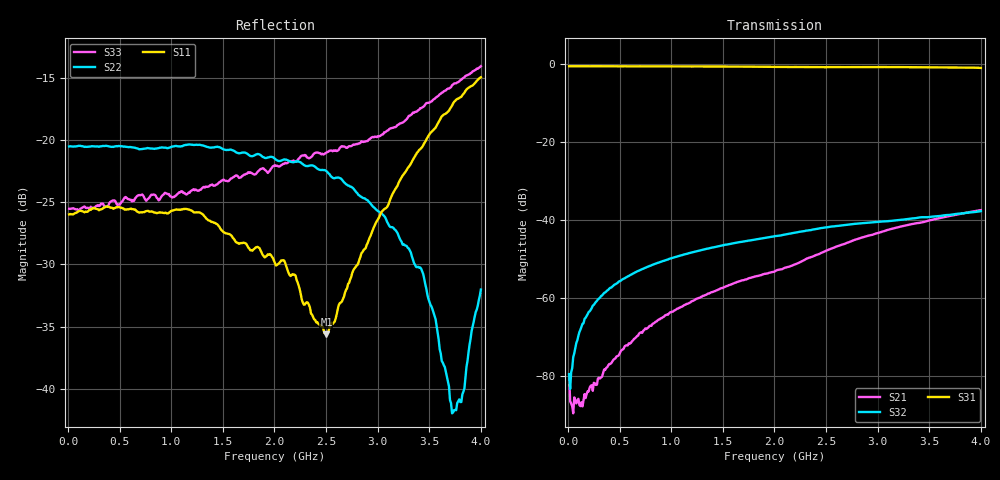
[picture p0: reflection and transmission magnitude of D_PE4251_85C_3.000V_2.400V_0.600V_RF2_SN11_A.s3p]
! Device ID: PE4251_SoldCshunt_081809
! Dir: c:\Test Bench Repositories\Bench_Software_CVI_Version_8\trunk\PSC 4Port_VNA Bench\datalog\4250\TEST\PE4251_SoldCshunt_081809\85C\3p000000\RF2
! Serial: 11
! Insertion: A
! Temp: 85C
! VDD: 3.000
! Control_Hi: 80.000
! Control_Lo: 20.000
! Logic State: RF2
! Port 1: RFC
! Port 2: RF1
! Port 3: RF2
! V1 = 0.60
! V2 = 0.60
! V3 = 0.60
! IDD: 4.342810e-05
! FILE NAME
! DATE 08/18/09  20:16
! CORRECTED  DATA
#  Hz  S  RI  R  50.00
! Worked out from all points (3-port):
!   401 points, 10 MHz to 4 GHz, reference 50 ohm
!   strongest paths, dB at 10 MHz, 1.008 GHz, 2.005 GHz, 3.002 GHz, 4 GHz:
!     S31: -0.6, -0.7, -0.8, -0.8, -1.1
!     S32: -79.4, -49.7, -44.1, -40.5, -37.7
!     S21: -79.6, -63.5, -53.1, -43.3, -37.5
!   lowest |S11| = -35.6 dB at 2.504 GHz (marker M1), VSWR 1.03, Z = 50.4 - j1.61 ohm
!   |S11| at or under -10 dB: start of sweep to end of sweep
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1e7  0.0502 -0.000826  9.81e-06 -2.35e-05  0.9306 -0.00374
     0.000105 6.75e-06  0.0942 -0.000936  2.63e-05 -3.63e-05
     0.931 -0.0045  1.43e-05 -0.000106  0.0529 0.000571
1.79575e8  0.0514 6.12e-05  7.43e-06 -5.77e-05  0.9288 -0.0635
           9.97e-06 -5.83e-05  0.0937 -0.00445  7.21e-05 0.00059
           0.9285 -0.0633  5.73e-05 0.00059  0.0533 -0.000987
3.19225e8  0.0526 -0.00155  -4.97e-05 -9.73e-05  0.9227 -0.1114
           -3.73e-05 -8.93e-05  0.0939 -0.00829  9.15e-05 0.00105
           0.9246 -0.1107  8.28e-05 0.00106  0.0554 -0.00304
4.888e8  0.0537 -0.00355  -0.000133 -0.00013  0.9126 -0.1684
         -0.000129 -0.000131  0.0938 -0.0121  0.000145 0.0016
         0.9129 -0.1676  0.000158 0.00161  0.0548 -0.00534
1.0075e9  0.0501 -0.0138  -0.000653 -0.000148  0.8626 -0.3352
          -0.000654 -0.000143  0.0902 -0.0264  0.000435 0.00324
          0.8638 -0.3354  0.000441 0.00325  0.0572 -0.0131
2.005e9  0.031 -0.00771  -0.00221 -6.32e-05  0.6873 -0.6014
         -0.00222 -4.25e-05  0.0772 -0.033  0.00103 0.00612
         0.6881 -0.6018  0.00102 0.00614  0.0691 -0.0387
2.50375e9  0.0046 -0.0159  -0.00404 -0.000364  0.5769 -0.6985
           -0.00406 -0.000383  0.0686 -0.0302  0.00136 0.00795
           0.579 -0.699  0.00137 0.00794  0.0514 -0.0727
3.42145e9  -0.0834 -0.0405  -0.00907 0.00198  0.3268 -0.8445
           -0.00907 0.00197  0.0244 -0.0182  0.00201 0.0106
           0.33 -0.844  0.002 0.0107  -0.0363 -0.1292
3.74065e9  -0.1364 -0.0407  -0.011 0.00352  0.2171 -0.8701
           -0.011 0.00351  -0.00112 -0.00814  0.00188 0.0117
           0.2175 -0.8701  0.00188 0.0117  -0.0921 -0.1412
4e9  -0.1757 -0.0322  -0.0125 0.0051  0.1214 -0.8779
     -0.0124 0.00506  -0.0249 -0.00302  0.00197 0.0128
     0.1233 -0.877  0.00192 0.0128  -0.1412 -0.1387
